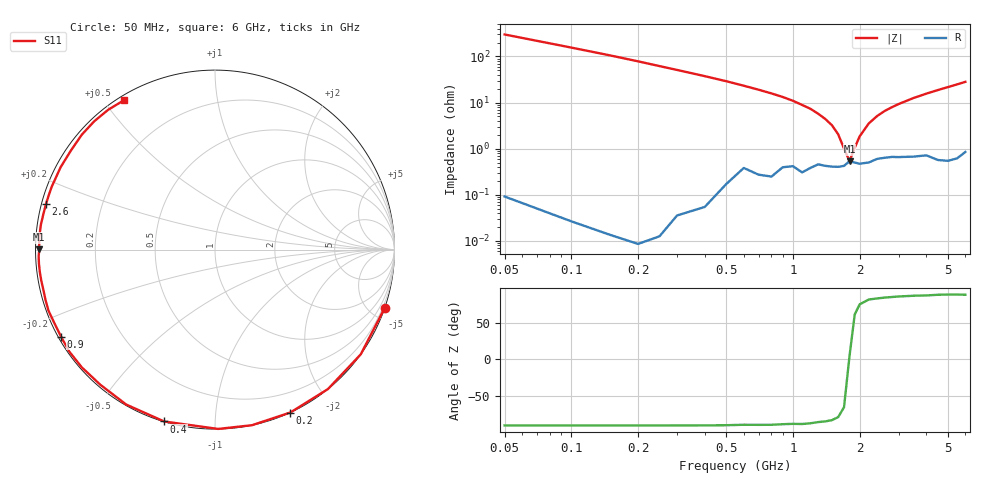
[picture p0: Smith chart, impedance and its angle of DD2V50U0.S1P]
! Infineon Technologies  Discrete & RF Semiconductors
! BBY58-02W
! Si Tuning Diode in SCD-80
! VR = 2.5 V
! S-Parameters:  June  2000
# GHz  S  MA  R  50
!  f  S11
! GHz  MAG  ANG
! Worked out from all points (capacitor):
!   34 points, 50 MHz to 6 GHz, reference 50 ohm
!   read as one part to ground: C = 10.2 pF near 50 MHz
!   lowest |Z| = 537 mohm at 1.8 GHz (marker M1)
!   series resonance near 1.795 GHz, so ESL is about 770 pH
!   S11 on the Smith chart (normalised r, x): 50 MHz: 0.00, -5.98; 200 MHz: 0.00, -1.56; 400 MHz: 0.00, -0.75; 900 MHz: 0.01, -0.26; 2.6 GHz: 0.01, +0.13; 6 GHz: 0.02, +0.56
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0.05  0.9999 -19.0
0.1  0.9999 -35.7
0.15  0.9999 -51.0
0.2  0.9999 -65.2
0.25  0.9998 -78.1
0.3  0.9993 -89.0
0.4  0.9986 -106.5
0.5  0.9949 -119.8
0.6  0.9875 -130.3
0.7  0.9905 -138.5
0.8  0.991 -145.0
0.9  0.9853 -150.5
1.1  0.9882 -159.9
1.3  0.9821 -167.0
1.4  0.9833 -170.0
1.6  0.984 -175.4
1.8  0.9788 179.9
2  0.9813 175.9
2.2  0.9802 172.0
2.4  0.9765 168.4
2.6  0.9753 165.0
3  0.9749 159.0
3.5  0.975 151.9
4  0.9742 145.4
4.5  0.9802 139.2
5  0.9818 133.3
5.5  0.9804 127.4
6  0.9745 121.3
